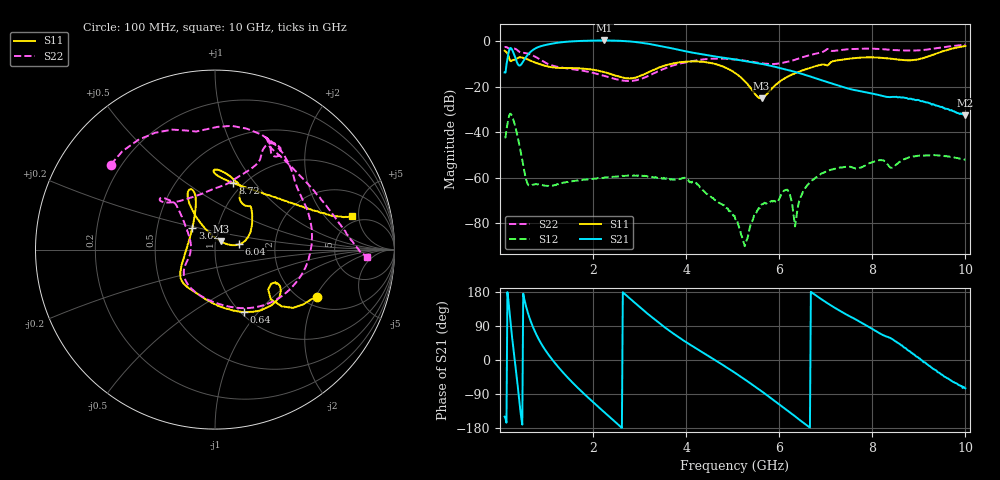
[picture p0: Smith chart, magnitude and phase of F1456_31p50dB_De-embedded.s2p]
! Integrated Device Technology
! Corporate Headquarters
! 6024 Silver Creek Valley Road
! San Jose, CA 95138  USA
! Phone:  1-408-284-8200
! Toll Free:  1-800-223-1366
! Webpage:  http://www.idt.com/
! Timing and RF Division
! 515 Groton Road, Suite 102
! Westford, MA 01886-6024
! Device:  F1456
! Description: 6-bit 0.5 dB Transmit Variable Gain Amplifier
! Frequency:  2100.0 -  2950.00 MHz
! Package:  6x6 mm Thin QFN Plastic Package: 28 pin
! State:  63
! Atten State:  31.5 dB
! Voltage:  +5.00 Volts
! Current:  216.902 mA
! Data:  The device was measured on a the F1455 evaluation board which has
!  individual transmission lines to the RF pins.  Data was collected
!  using a calibrated network analyzer.  The evaluation board was
!  de-embedded using a TRL calibration technique.
!  The reference plane is the edge of the package pin.
!  Pin  1 = CSb
!  Pin  2 = DATA
!  Pin  3 = CLK
!  Pin  4 = RSET
!  Pin  5 = GND
!  Pin  6 = RFIN  = Port 1
!  Pin  7 = GND
!  Pin  8 = NC
!  Pin  9 = NC
!  Pin 10 = NC
!  Pin 11 = NC
!  Pin 12 = NC
!  Pin 13 = NC
!  Pin 14 = /STBY
!  Pin 15 = GND
!  Pin 16 = RFOUT  = Port 2
!  Pin 17 = GND
!  Pin 18 = NC
!  Pin 19 = NC
!  Pin 20 = NC
!  Pin 21 = GND
!  Pin 22 = NC
!  Pin 23 = GND
!  Pin 24 = NC
!  Pin 25 = NC
!  Pin 26 = NC
!  Pin 27 = GND
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# GHz S dB R 50
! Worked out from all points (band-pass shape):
!   496 points, 100 MHz to 10 GHz, reference 50 ohm
!   highest |S21| = 0.40 dB at 2.24 GHz (marker M1); lowest = -32.5 dB at 10 GHz (marker M2)
!   |S21| within 3 dB of the highest: 812.8 MHz to 3.584 GHz (2.772 GHz wide, 126 % of centre)
!   lowest |S11| = -25.0 dB at 5.62 GHz (marker M3), VSWR 1.12, Z = 53.1 + j4.87 ohm
!   |S11| at or under -10 dB: 846.8 MHz to 3.657 GHz (2.81 GHz wide, 125 % of centre); 4.633 GHz to 7.072 GHz (2.439 GHz wide, 41.7 % of centre)
!   |S22| runs from -17.4 to -1.5 dB; largest |S21 - S12| = 1
!   S11 on the Smith chart (normalised r, x): 100 MHz: 2.37, -2.04; 640 MHz: 1.03, -0.84; 3.02 GHz: 0.76, +0.19; 6.04 GHz: 1.31, +0.08; 8.72 GHz: 0.90, +0.78; 10 GHz: 4.19, +4.18
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0.1  -4.10 -24.9  -13.68 -149.5  -42.28 50.5  -2.51 140.7
0.18  -6.24 -40.4  -5.43 159.9  -34.14 -2.4  -2.98 109.6
0.26  -8.35 -28.4  -3.65 60.7  -32.88 -101.1  -3.30 88.8
0.4  -7.16 -33.7  -10.46 -90.0  -43.82 149.5  -4.35 44.3
0.64  -8.32 -65.1  -4.96 109.4  -63.44 135.1  -5.62 -6.5
0.82  -9.82 -83.2  -2.53 57.9  -62.86 119.8  -7.48 -45.2
1.14  -11.46 -109.4  -0.92 -1.6  -63.39 90.5  -10.73 -92.6
1.76  -11.92 -137.5  0.21 -83.8  -61.01 58.6  -12.83 -138.8
2.24  -13.53 -153.1  0.40 -137.6  -59.90 43.4  -15.15 -155.8
2.62  -15.88 -178.6  0.21 -179.1  -59.18 30.1  -17.20 -172.8
3.02  -15.15 136.5  -0.55 137.8  -59.35 13.3  -16.51 159.1
3.4  -11.67 114.4  -1.84 99.4  -59.84 -1.1  -13.21 139.9
4.12  -8.79 112.3  -4.90 37.9  -62.14 -35.8  -8.73 132.2
5.06  -13.98 119.7  -7.97 -34.7  -78.31 -55.5  -7.97 138.0
5.62  -25.05 54.8  -9.92 -82.3  -71.77 106.4  -9.64 123.4
6.04  -17.25 12.3  -11.86 -120.8  -67.54 103.9  -9.56 94.2
6.2  -15.32 15.8  -12.70 -135.3  -66.14 63.6  -8.87 82.8
6.34  -14.02 21.2  -13.41 -148.6  -81.40 90.3  -8.08 76.2
6.7  -11.44 39.5  -15.67 178.1  -61.30 128.2  -5.83 64.9
8.36  -7.53 89.5  -24.49 59.3  -54.94 46.1  -3.72 62.4
8.72  -8.31 74.7  -24.87 30.9  -51.54 57.5  -4.02 50.2
10  -2.06 13.8  -32.53 -74.8  -52.00 -32.3  -1.46 -2.6
